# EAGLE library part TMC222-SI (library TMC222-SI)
Micro Stepping Stepper Motor Controller / Driver with Two Wire Serial Interface, SO20
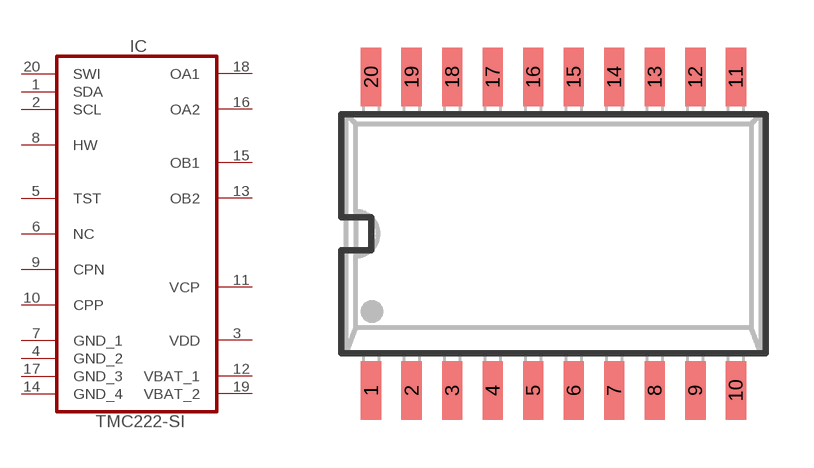
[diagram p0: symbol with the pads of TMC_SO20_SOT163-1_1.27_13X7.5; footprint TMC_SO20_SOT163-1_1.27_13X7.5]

Designator prefix IC

## TMC222-SI (DATASHEET: http://www_trinamic_com/_scripts/download_php?file=_articles%2Fproducts%2Fintegrated-circuits%2Ftmc222%2F_datasheet%2FTMC222_datasheet_pdf; DESCRIPTION: Micro Stepping Stepper Motor Controller / Driver with Two Wire Serial Interface, SO20; DISTRIBUTOR1: Digikey; DISTRIBUTOR2: Farnell; GEOMETRY_HEIGHT: 2,65mm; MANUFACTURER: TRINAMIC; ORDERCODE-DISTRI1: 1460-1052-5-ND; ORDERCODE-DISTRI2: 1214195; ORDERCODE-MANU1: TMC222-SI; VALUE: TMC222-SI)  [TMC_SO20_SOT163-1_1.27_13X7.5]
1  SDA
2  SCL  in
3  VDD  pwr
4  GND_2  pwr
5  TST  in
6  NC  pas
7  GND_1  pwr
8  HW  in
9  CPN
10  CPP
11  VCP  pwr
12  VBAT_1  pwr
13  OB2  out
14  GND_4  pwr
15  OB1  out
16  OA2  out
17  GND_3  pwr
18  OA1  out
19  VBAT_2  pwr
20  SWI  in

## Footprint TMC_SO20_SOT163-1_1.27_13X7.5 (pad centres in mm)
smd 0.64 x 1.83: 1 -5.715,-4.912; 2 -4.445,-4.912; 3 -3.175,-4.912; 4 -1.905,-4.912; 5 -0.635,-4.912; 6 0.635,-4.912; 7 1.905,-4.912; 8 3.175,-4.912; 9 4.445,-4.912; 10 5.715,-4.912; 11 5.715,4.912; 12 4.445,4.912; 13 3.175,4.912; 14 1.905,4.912; 15 0.635,4.912; 16 -0.635,4.913; 17 -1.905,4.912; 18 -3.175,4.912; 19 -4.445,4.912; 20 -5.715,4.912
